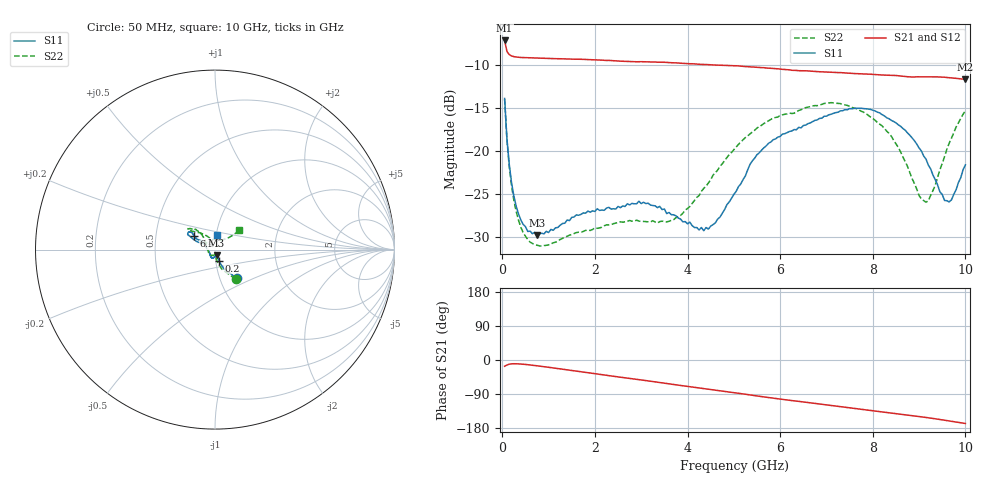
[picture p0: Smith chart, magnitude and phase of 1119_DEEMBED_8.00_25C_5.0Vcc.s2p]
!Hittite Microwave Corp.
!Digital Attenuator/PhaseShifter Rev 1.4.0
!Filename: C:\DATA\DATA\1119_DEEMBED_8.00_25C_5.0Vcc.s2p
!VNA ID: Agilent Technologies,N5224A,MY51441122,A.10.45.03
!Device type:
!2 Port Calibration.
!Temp(C): 25
!Lot Number:
!Serial Number:
!Operator:
!Misc:
!Attenuator:  8.000
# GHZ S DB R 50.0
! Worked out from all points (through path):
!   200 points, 50 MHz to 10 GHz, reference 50 ohm
!   highest |S21| = -7.14 dB at 50 MHz (marker M1); lowest = -11.7 dB at 10 GHz (marker M2)
!   group delay of S21, straight-line fit = 45.1 ps
!   lowest |S11| = -29.8 dB at 750 MHz (marker M3), VSWR 1.07, Z = 50.8 - j3.18 ohm
!   |S11| at or under -10 dB: start of sweep to end of sweep
!   |S22| runs from -31.1 to -13.9 dB; largest |S21 - S12| = 0.0031
!   S11 on the Smith chart (normalised r, x): 50 MHz: 1.21, -0.40; 200 MHz: 1.04, -0.13; 6.4 GHz: 0.79, +0.12; 10 GHz: 1.01, +0.17
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0.05  -13.89 -52.6  -7.14 -16.5  -7.14 -16.5  -13.95 -55.3
0.1  -18.56 -65.2  -8.41 -13.3  -8.40 -13.3  -18.68 -70.5
0.2  -23.72 -69.8  -8.94 -10.2  -8.94 -10.2  -24.05 -80.0
0.4  -28.03 -69.5  -9.12 -10.6  -9.12 -10.6  -28.87 -85.2
0.75  -29.77 -74.3  -9.20 -15.3  -9.19 -15.3  -30.97 -90.6
1.75  -27.21 -96.0  -9.34 -31.8  -9.34 -31.8  -29.36 -108.3
2.95  -25.85 -109.7  -9.61 -51.7  -9.61 -51.8  -28.16 -145.6
3.4  -26.45 -120.2  -9.67 -59.4  -9.67 -59.4  -28.22 -165.9
3.85  -27.93 -132.4  -9.79 -67.2  -9.78 -67.2  -27.50 170.6
4.35  -29.28 -156.4  -9.93 -75.3  -9.94 -75.4  -24.36 145.8
5.05  -24.70 159.4  -10.10 -86.8  -10.11 -86.8  -19.51 131.7
5.5  -20.43 148.7  -10.27 -94.9  -10.24 -94.6  -17.33 132.8
6.4  -17.25 147.3  -10.66 -109.2  -10.65 -108.7  -15.29 138.3
6.7  -16.59 145.5  -10.72 -113.8  -10.71 -113.3  -14.76 139.9
7.65  -15.03 147.3  -11.00 -128.5  -10.98 -127.9  -15.07 142.7
8.35  -16.25 152.5  -11.18 -139.3  -11.15 -139.3  -17.94 132.1
8.7  -17.58 154.5  -11.34 -145.0  -11.32 -144.9  -21.23 120.1
8.999999  -19.66 156.3  -11.37 -149.3  -11.38 -149.2  -25.19 100.5
9.15  -20.95 155.3  -11.37 -151.6  -11.38 -151.6  -25.97 82.2
9.45  -24.77 141.8  -11.39 -157.0  -11.40 -156.9  -22.19 48.0
9.65  -25.93 114.0  -11.47 -160.8  -11.47 -160.7  -19.10 40.3
10  -21.62 80.4  -11.67 -167.5  -11.67 -167.5  -15.32 39.0
